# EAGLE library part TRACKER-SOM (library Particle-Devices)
Particle Tracker SoM Tracker SoM is a powerful, configurable, and extensible IoT System-on-Module (SoM) that builds on Particle's Tracking Services foundation and provides a powerful MCU, GNSS, and advanced peripherals in a compact form factor. More information: https://docs.particle.io/datasheets/asset-tracking/tracker-som-datasheet/
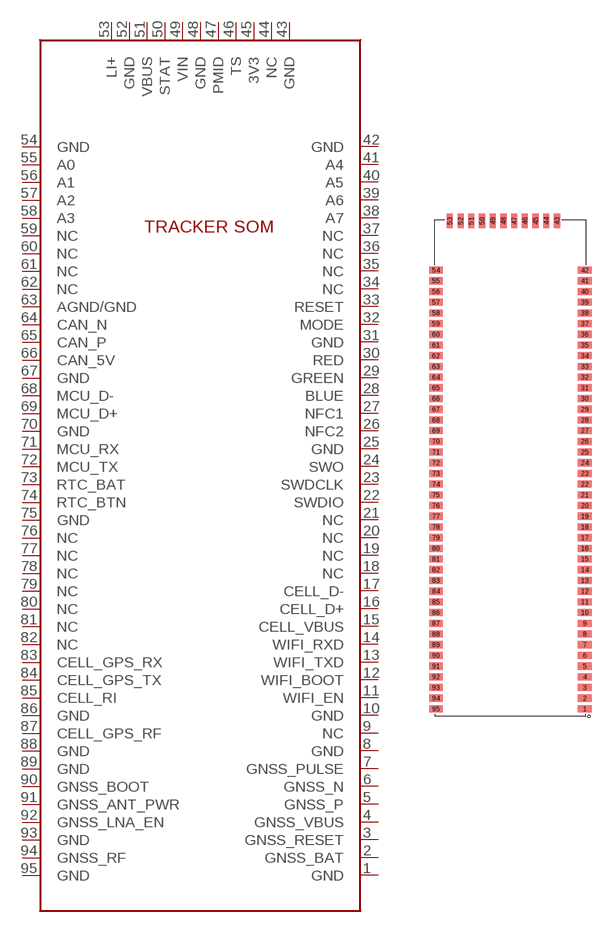
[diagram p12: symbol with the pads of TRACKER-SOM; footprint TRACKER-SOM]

Designator prefix U

## TRACKER-SOM  [TRACKER-SOM]
1  GND
2  GNSS_BAT
3  GNSS_RESET
4  GNSS_VBUS
5  GNSS_P
6  GNSS_N
7  GNSS_PULSE
8  GND
9  NC
10  GND
11  WIFI_EN
12  WIFI_BOOT
13  WIFI_TXD
14  WIFI_RXD
15  CELL_VBUS
16  CELL_D+
17  CELL_D-
18  NC
19  NC
20  NC
21  NC
22  SWDIO
23  SWDCLK
24  SWO
25  GND
26  NFC2
27  NFC1
28  BLUE
29  GREEN
30  RED
31  GND
32  MODE
33  RESET
34  NC
35  NC
36  NC
37  NC
38  A7
39  A6
40  A5
41  A4
42  GND
43  GND
44  NC
45  3V3
46  TS
47  PMID
48  GND
49  VIN
50  STAT
51  VBUS
52  GND
53  LI+
54  GND
55  A0
56  A1
57  A2
58  A3
59  NC
60  NC
61  NC
62  NC
63  AGND/GND
64  CAN_N
65  CAN_P
66  CAN_5V
67  GND
68  MCU_D-
69  MCU_D+
70  GND
71  MCU_RX
72  MCU_TX
73  RTC_BAT
74  RTC_BTN
75  GND
76  NC
77  NC
78  NC
79  NC
80  NC
81  NC
82  NC
83  CELL_GPS_RX
84  CELL_GPS_TX
85  CELL_RI
86  GND
87  CELL_GPS_RF
88  GND
89  GND
90  GNSS_BOOT
91  GNSS_ANT_PWR
92  GNSS_LNA_EN
93  GND
94  GNSS_RF
95  GND

## Footprint TRACKER-SOM (pad centres in mm)
smd 2.8 x 1.35: 1 27.9,-91.3; 2 27.9,-89.3; 3 27.9,-87.3; 4 27.9,-85.3; 5 27.9,-83.3; 6 27.9,-81.3; 7 27.9,-79.3; 8 27.9,-77.3; 9 27.9,-75.3; 10 27.9,-73.3; 11 27.9,-71.3; 12 27.9,-69.3; 13 27.9,-67.3; 14 27.9,-65.3; 15 27.9,-63.3; 16 27.9,-61.3; 17 27.9,-59.3; 18 27.9,-57.3; 19 27.9,-55.3; 20 27.9,-53.3; 21 27.9,-51.3; 22 27.9,-49.3; 23 27.9,-47.3; 24 27.9,-45.3; 25 27.9,-43.3; 26 27.9,-41.3; 27 27.9,-39.3; 28 27.9,-37.3; 29 27.9,-35.3; 30 27.9,-33.3; 31 27.9,-31.3; 32 27.9,-29.3; 33 27.9,-27.3; 34 27.9,-25.3; 35 27.9,-23.3; 36 27.9,-21.3; 37 27.9,-19.3; 38 27.9,-17.3; 39 27.9,-15.3; 40 27.9,-13.3; 41 27.9,-11.3; 42 27.9,-9.3; 54 0.1,-9.3; 55 0.1,-11.3; 56 0.1,-13.3; 57 0.1,-15.3; 58 0.1,-17.3; 59 0.1,-19.3; 60 0.1,-21.3; 61 0.1,-23.3; 62 0.1,-25.3; 63 0.1,-27.3; 64 0.1,-29.3; 65 0.1,-31.3; 66 0.1,-33.3; 67 0.1,-35.3; 68 0.1,-37.3; 69 0.1,-39.3; 70 0.1,-41.3; 71 0.1,-43.3; 72 0.1,-45.3; 73 0.1,-47.3; 74 0.1,-49.3; 75 0.1,-51.3; 76 0.1,-53.3; 77 0.1,-55.3; 78 0.1,-57.3; 79 0.1,-59.3; 80 0.1,-61.3; 81 0.1,-63.3; 82 0.1,-65.3; 83 0.1,-67.3; 84 0.1,-69.3; 85 0.1,-71.3; 86 0.1,-73.3; 87 0.1,-75.3; 88 0.1,-77.3; 89 0.1,-79.3; 90 0.1,-81.3; 91 0.1,-83.3; 92 0.1,-85.3; 93 0.1,-87.3; 94 0.1,-89.3; 95 0.1,-91.3
smd 1.35 x 2.8: 43 22.7,-0.1; 44 20.7,-0.1; 45 18.7,-0.1; 46 16.7,-0.1; 47 14.7,-0.1; 48 12.7,-0.1; 49 10.7,-0.1; 50 8.7,-0.1; 51 6.7,-0.1; 52 4.7,-0.1; 53 2.7,-0.1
